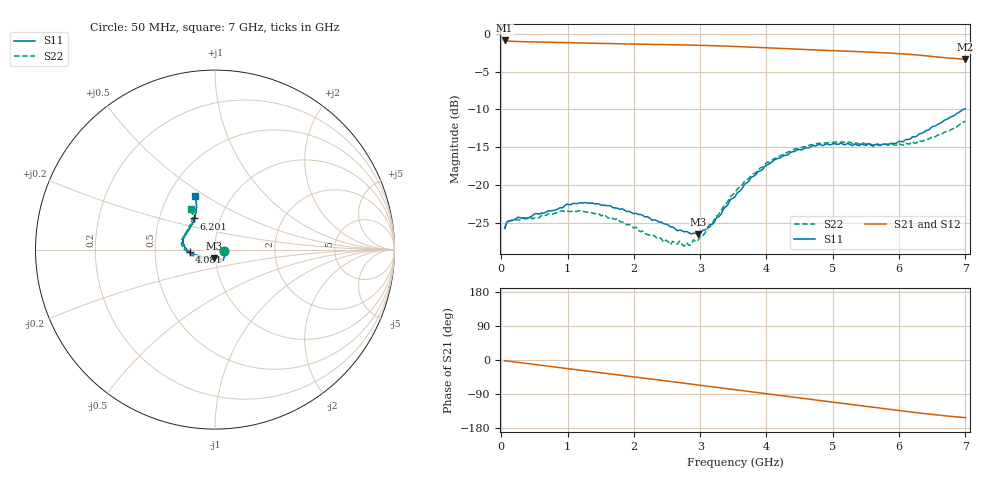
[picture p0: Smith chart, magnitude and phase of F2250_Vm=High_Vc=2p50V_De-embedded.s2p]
! Integrated Device Technology
! Corporate Headquarters
! 6024 Silver Creek Valley Road
! San Jose, CA 95138  USA
! Phone:  1-408-284-8200
! Toll Free:  1-800-223-1366
! Webpage:  http://www.idt.com/
! Timing and RF Division
! 515 Groton Road, Suite 102
! Westford, MA 01886-6024
! Device:  F2250
! Description: Voltage Variable RF Attenuator
! Frequency:  50.0 -  6000.00 MHz
! Package:  3x3 mm Thin QFN Plastic Package: 16 pin
! Ports:  2 RF, 3 DC
!  Pin  1  = GND
!  Pin  2  = NC
!  Pin  3  = RF1  = Port 1
!  Pin  4  = NC
!  Pin  5  = GND
!  Pin  6  = GND
!  Pin  7  = GND
!  Pin  8  = GND
!  Pin  9  = NC
!  Pin 10  = RF2  = Port 2
!  Pin 11  = NC
!  Pin 12  = GND
!  Pin 13  = GND
!  Pin 14  = VCNTRL
!  Pin 15  = VDD
!  Pin 16  = VMODE
! Vcntrl:  2.500 Volts
! Vmode:  +3.300 Volts
! Vdd:  +3.30  Volts
! Current:  1.313 mA
! Data:  The device was measured on a the F2250 evaluation board which has
!  individual transmission lines to the RF pins.  Data was collected
!  using a calibrated network analyzer.  The evaluation board was
!  de-embedded using a TRL calibration technique.
!  The reference plane is the edge of the package pin.
! Misc:  SN 10
!  Action Tracker AT0258
! Date Measured:  2014-11-26
! Date:  2015-10-15  MJV
! Note:
!  Integrated Device Technology supplies this data as a sample of measured
!  data at the package pin for this product.  Your particular data for this
!  product may vary.
!  Data was taken at 25 degrees C.
!  Integrated Device Technology reserves the right to change this data at anytime.
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# GHz S dB R 50
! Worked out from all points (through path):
!   201 points, 50 MHz to 7 GHz, reference 50 ohm
!   highest |S21| = -0.89 dB at 50 MHz (marker M1); lowest = -3.4 dB at 7 GHz (marker M2)
!   group delay of S21, straight-line fit = 61.2 ps
!   lowest |S11| = -26.5 dB at 2.969 GHz (marker M3), VSWR 1.10, Z = 49.1 - j4.62 ohm
!   |S11| at or under -10 dB: start of sweep to 6.967 GHz
!   |S22| runs from -28.1 to -11.6 dB; largest |S21 - S12| = 0.0019
!   S11 on the Smith chart (normalised r, x): 50 MHz: 1.11, -0.02; 4.081 GHz: 0.75, -0.02; 6.201 GHz: 0.75, +0.27; 7 GHz: 0.68, +0.45
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0.05  -25.65 -10.7  -0.89 -1.8  -0.89 -1.8  -25.81 -10.9
0.1195  -24.75 -10.2  -0.98 -3.2  -0.98 -3.2  -24.68 -8.9
0.57125  -23.83 -31.3  -1.10 -13.3  -1.10 -13.3  -24.33 -31.4
0.91875  -23.00 -50.1  -1.17 -21.0  -1.17 -21.1  -23.36 -51.0
1.2315  -22.36 -57.9  -1.24 -27.9  -1.24 -27.9  -23.47 -61.6
1.75275  -23.04 -64.9  -1.33 -39.1  -1.33 -39.1  -24.42 -67.8
2.37825  -24.87 -64.5  -1.42 -52.8  -1.42 -52.8  -26.86 -66.8
2.552  -25.51 -69.5  -1.44 -56.7  -1.44 -56.7  -27.85 -73.2
2.691  -25.93 -77.5  -1.47 -59.8  -1.47 -59.8  -27.38 -80.9
2.7605  -26.17 -79.7  -1.48 -61.3  -1.48 -61.3  -28.05 -85.4
2.969  -26.49 -97.8  -1.52 -66.0  -1.52 -66.0  -27.28 -105.0
3.1775  -25.20 -120.8  -1.57 -70.7  -1.57 -70.7  -25.24 -126.9
3.525  -21.54 -152.8  -1.68 -78.5  -1.68 -78.6  -20.97 -148.8
3.76825  -18.96 -164.8  -1.77 -84.0  -1.77 -84.1  -18.70 -159.7
4.081  -16.95 -175.7  -1.90 -91.0  -1.90 -91.0  -16.72 -171.5
4.4285  -15.54 176.0  -2.03 -98.6  -2.04 -98.7  -15.20 178.6
4.7065  -14.76 169.1  -2.13 -104.8  -2.13 -104.8  -14.69 172.9
5.054  -14.61 160.9  -2.26 -112.5  -2.26 -112.5  -14.29 165.9
5.85325  -14.57 135.1  -2.56 -130.0  -2.56 -130.1  -14.69 147.2
6.20075  -13.62 123.6  -2.77 -137.7  -2.77 -137.8  -14.27 138.2
6.54825  -12.18 115.6  -3.04 -144.7  -3.04 -144.9  -13.60 126.9
7  -9.91 110.8  -3.37 -152.1  -3.38 -152.2  -11.56 120.6
